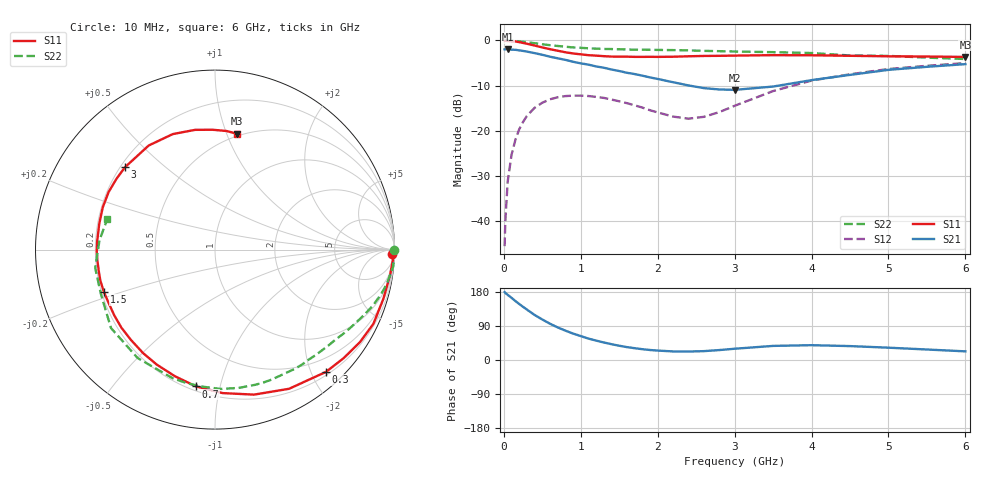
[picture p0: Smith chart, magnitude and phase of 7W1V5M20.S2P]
! Infineon Technologies  Discrete & RF Semiconductors
! BFS17W
! Si NPN RF Bipolar Junction Transistor in SOT323
! VCE = 1.5 V  IC = 0.2 mA
! Common Emitter S-Parameters:  August  1999
# GHz  S  MA  R  50
!  f  S11  S21  S12  S22
! GHz  MAG  ANG  MAG  ANG  MAG  ANG  MAG  ANG
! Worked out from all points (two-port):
!   36 points, 10 MHz to 6 GHz, reference 50 ohm
!   highest |S21| = -1.93 dB at 50 MHz (marker M1); lowest = -10.9 dB at 3 GHz (marker M2)
!   |S21| within 3 dB of the highest: start of sweep to 960.1 MHz
!   lowest |S11| = -3.6 dB at 6 GHz (marker M3), VSWR 4.83, Z = 24 + j54.4 ohm
!   |S11| at or under -10 dB: nowhere
!   |S22| runs from -4.1 to 0.0 dB; largest |S21 - S12| = 0.8
!   S11 on the Smith chart (normalised r, x): 10 MHz: 28, -64; 300 MHz: 0.25, -2.23; 700 MHz: 0.23, -0.85; 1.5 GHz: 0.21, -0.18; 3 GHz: 0.22, +0.37; 6 GHz: 0.48, +1.09
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0.01  0.9887 -1.5  0.798 179.3  0.0053 89.6  0.9999 -0.1
0.02  0.9926 -3.5  0.798 176.9  0.0103 88.7  0.9968 -1.1
0.05  0.9855 -8.3  0.801 171.9  0.0275 86.0  0.9977 -2.7
0.1  0.9774 -16.3  0.791 164.1  0.0543 79.5  0.9966 -5.5
0.15  0.9746 -25.1  0.788 155.6  0.0795 73.6  0.9868 -8.1
0.2  0.9582 -32.5  0.777 147.8  0.1041 69.3  0.9779 -10.6
0.3  0.92 -47.8  0.753 133.0  0.1463 59.3  0.9562 -15.4
0.4  0.8784 -62.0  0.724 118.9  0.18 50.6  0.9322 -19.7
0.5  0.8369 -74.9  0.694 106.9  0.2047 42.9  0.9079 -23.5
0.7  0.7695 -97.9  0.635 86.0  0.2352 30.6  0.8687 -30.5
0.9  0.7183 -116.8  0.581 69.7  0.2451 20.9  0.8374 -36.9
1.1  0.6874 -133.0  0.54 56.5  0.2428 13.8  0.819 -43.2
1.5  0.6626 -159.1  0.459 37.6  0.2123 5.2  0.7995 -56.1
2.2  0.6608 167.3  0.345 22.6  0.1438 15.4  0.7818 -80.3
2.6  0.6739 151.7  0.297 23.4  0.1429 38.0  0.7671 -94.6
3  0.6798 137.6  0.284 29.7  0.1892 53.2  0.7545 -108.2
3.5  0.6876 122.5  0.309 37.2  0.2755 56.4  0.7422 -125.5
4  0.6852 110.1  0.364 39.1  0.3598 51.3  0.7258 -143.0
4.5  0.6764 99.5  0.416 36.7  0.4226 44.5  0.6823 -158.6
5  0.6679 91.3  0.473 32.5  0.4833 37.8  0.6752 -171.3
5.5  0.664 84.6  0.511 27.7  0.5243 31.4  0.6456 175.3
6  0.657 79.2  0.547 22.8  0.5623 25.5  0.6235 164.0
